(* Logix 5000 Routine export IS7800_Job_Change; software revision 33.01 *)

VAR_GLOBAL   (* controller tags *)
   Camera_JobName : STRING := '3_Test.job';
   IS7800_Job_Change : BOOL;
   IS7800_Job_Change_MSG : MESSAGE;
        MessageParameters(MessageType := CIP Generic, RequestedLength := 32, ConnectedFlag := 2, ConnectionPath := IS7800, ServiceCode := 16#0010, ObjectType := 16#0078, TargetObject := 1, AttributeNumber := 16#0014, LocalElement := SetJobData[0])
   SetJobData : SINT[32] := ([0] := 10, [2] := 51, [3] := 95, [4] := 84, [5] := 101, [6] := 115, [7] := 116, [8] := 46, [9] := 106, [10] := 111, [11] := 98);
END_VAR

PROGRAM MainProgram

ROUTINE IS7800_Job_Change   (* ladder *)
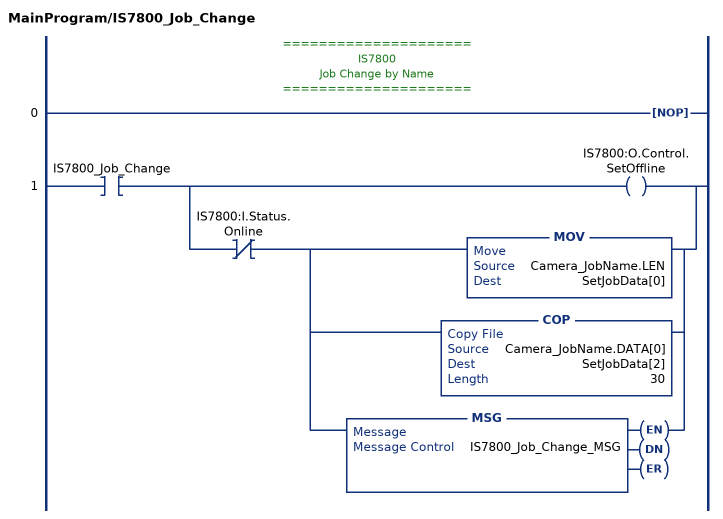
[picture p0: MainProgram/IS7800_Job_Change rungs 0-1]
   // =====================
   // IS7800
   // Job Change by Name
   // =====================
   0: NOP();
   1: XIC(IS7800_Job_Change)[OTE(IS7800:O.Control.SetOffline) ,XIO(IS7800:I.Status.Online) [MOV(Camera_JobName.LEN,SetJobData[0]) ,COP(Camera_JobName.DATA[0],SetJobData[2],30) ,MSG(IS7800_Job_Change_MSG) ] ];
END_ROUTINE
END_PROGRAM
